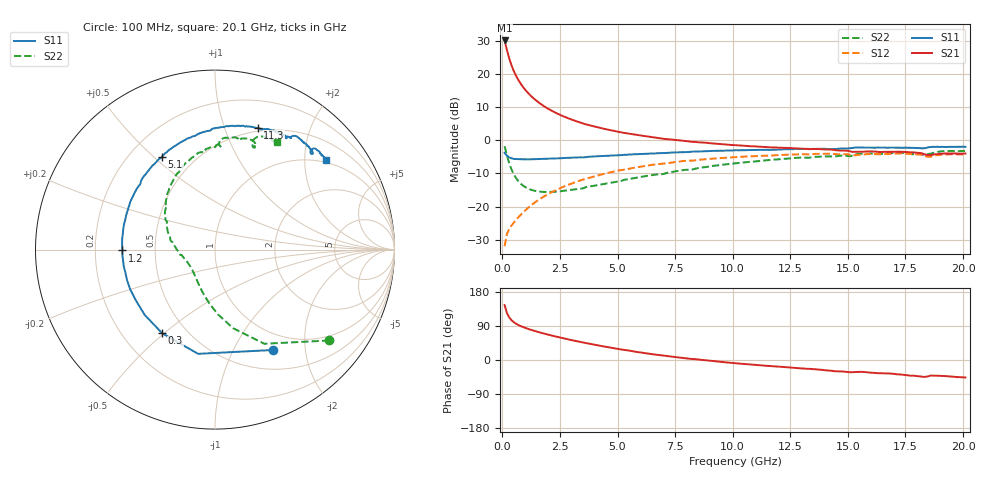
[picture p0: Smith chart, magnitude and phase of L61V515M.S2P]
!  Infineon Technologies AG
! BFR380L3 , PF131585-7, No.6, Th 09.10.01, soldered on pcb-board, measured with PP GSG850
!  Vce=1.5 V,  Ic=15.0 mA
! Common Emitter S-Parameters:  15. November 2001
#  GHz  S  MA  R  50
! f  S11  S21  S12  S22
! GHz  Mag  Ang  Mag  Ang  Mag  Ang  Mag  Ang
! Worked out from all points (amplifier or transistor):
!   201 points, 100 MHz to 20.1 GHz, reference 50 ohm
!   highest |S21| = 30.1 dB at 100 MHz (marker M1)
!   |S21| within 3 dB of that: start of sweep to 205.2 MHz
!   unconditionally stable (mu >= 1): 1.514 GHz to 4.71 GHz
!   at 3.4 GHz: K = 1.03, MAG = 7.7 dB, |S12| = -12.1 dB
!   at 10.1 GHz: K = 0.96, MSG = 1.8 dB, |S12| = -5.1 dB
!   at 20.1 GHz: K = 0.99, MSG = 0.1 dB, |S12| = -4.2 dB
!   S11 on the Smith chart (normalised r, x): 100 MHz: 0.76, -1.45; 300 MHz: 0.37, -0.49; 1.2 GHz: 0.32, -0.00; 5.1 GHz: 0.33, +0.53; 11.3 GHz: 0.46, +1.30; 20.1 GHz: 0.93, +2.54
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0.1  0.6462 -59.9  31.96 144.9  0.02536 64.9  0.8129 -38.5
0.2  0.5883 -99.2  22.97 124.0  0.03857 53.9  0.592 -62.4
0.3  0.5513 -122.2  17.14 112.5  0.04602 51.0  0.45 -77.0
0.4  0.5347 -137.1  13.49 105.0  0.0519 50.9  0.3624 -87.2
0.5  0.5239 -147.1  11.04 99.7  0.05743 52.5  0.3063 -95.2
0.6  0.5216 -154.8  9.323 95.7  0.06329 53.8  0.2684 -101.8
0.7  0.5191 -160.6  8.077 92.4  0.06935 55.4  0.2416 -107.6
0.8  0.5153 -165.6  7.112 89.5  0.07533 56.7  0.2219 -112.6
0.9  0.5167 -169.7  6.353 87.0  0.08162 57.6  0.2072 -117.0
1  0.5159 -173.2  5.748 84.6  0.08805 58.5  0.1966 -121.2
1.2  0.5163 -179.5  4.826 80.4  0.1013 59.7  0.182 -128.3
1.6  0.5208 170.8  3.667 73.2  0.1281 60.5  0.1688 -139.6
2.1  0.5276 160.9  2.841 65.2  0.1622 59.7  0.1672 -150.2
2.7  0.5413 151.0  2.26 56.6  0.2026 57.4  0.1741 -160.6
3.5  0.5529 139.1  1.796 46.1  0.2557 53.1  0.1886 -170.7
5.1  0.5956 119.7  1.331 28.2  0.3537 42.7  0.2409 169.8
6.8  0.6395 102.2  1.08 12.9  0.4401 31.3  0.3075 150.6
10.1  0.7067 77.7  0.8447 -8.3  0.5568 10.0  0.4499 121.6
11.3  0.7187 70.7  0.7979 -14.4  0.585 2.4  0.4942 111.8
13.5  0.7423 60.2  0.7393 -24.3  0.619 -10.4  0.5569 95.7
16.8  0.7753 48.1  0.6702 -35.6  0.6233 -25.9  0.6395 75.7
20.1  0.7961 38.8  0.6319 -46.2  0.617 -39.3  0.6917 60.1
